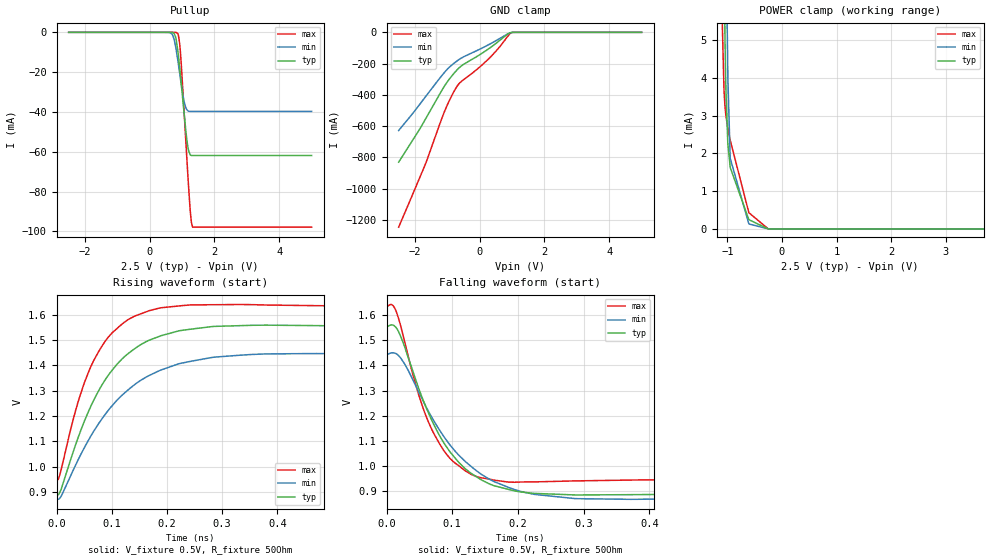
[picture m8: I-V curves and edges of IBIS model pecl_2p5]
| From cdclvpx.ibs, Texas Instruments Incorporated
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|   Pecl_2p5 Model   |
[Model]   pecl_2p5
Model_type   Open_source
Polarity   Non-Inverting
Vmeas = 1.22
Vref = 0.5
Cref = 1pF
Rref = 50
|   typ   min   max
|   (nom PVT)   (fast PVT)   (slow PVT)
C_comp   1.172e-13   1.121e-13   1.238e-13
[Model Spec]
|Subparameter
Vmeas   1.22V   1.16V   1.3V
| Vmeas is the expected cross point for each differential signal pair.
| Where nom  PVT is Nominal Process, 2.5V, 40C
|   Fast PVT is Strong Process,  2.625V, -40C
|   Slow PVT is Weak Process,   2.375V,100C
[Voltage Range]   2.5   2.375   2.625
|Junction Temperature
[Temperature range]   40   100   -40
[Pullup Reference]   2.5   2.375   2.625
[Pulldown Reference]   0   0   0
[Power Clamp Reference]   2.5   2.375   2.625
[GND Clamp Reference]   0   0   0
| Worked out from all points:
|   falling waveform, V_fixture 0.5V, R_fixture 50Ohm: 20-80 % time 72.8ps typ, 91.4ps min, 54.2ps max; typ from 1.55 V to 0.89 V
|   rising waveform, V_fixture 0.5V, R_fixture 50Ohm: 20-80 % time 91.7ps typ, 114ps min, 69.7ps max; typ from 0.89 V to 1.55 V
[GND Clamp]
|   Voltage   I(typ)   I(min)   I(max)
-2.5V     -829.8mA   -627.6mA   -1.246A
-1.827V   -610.9mA   -454.4mA   -917.9mA
-1.655V   -548.5mA   -407.4mA   -833.1mA
-1.09V    -345.1mA   -257.2mA   -508.6mA
-932.9mV  -298.3mA   -222.7mA   -434.9mA
-770mV    -256.8mA   -194.2mA   -369.5mA
-621.4mV  -224.8mA   -171.9mA   -324.6mA
-79.75mV  -153.8mA   -116.3mA   -236.2mA
352.4mV   -94.38mA   -70.87mA   -154mA
950mV     -2.212mA   -3.472mA   -5.936mA
1.078V    -34.58uA   -148.2uA   -28.47uA
5V        0A         0A         0A
[Pullup]
|   Voltage   I(typ)   I(min)   I(max)
-2.5V     0A         0A         0A
650mV     -16.5uA    -287.6uA   -23.75nA
799.6mV   -2.244mA   -6.925mA   -26.92uA
870mV     -9.197mA   -14.07mA   -689.7uA
928.3mV   -17.88mA   -20.73mA   -5.854mA
950.9mV   -21.58mA   -23.37mA   -10.13mA
1.06V     -40mA      -34.6mA    -38.68mA
1.167V    -56.25mA   -39.23mA   -68.43mA
1.251V    -61.52mA   -39.72mA   -89.32mA
1.288V    -61.88mA   -39.72mA   -95.39mA
1.33V     -61.88mA   -39.72mA   -97.87mA
5V        -61.88mA   -39.72mA   -97.87mA
[POWER Clamp]
|   Voltage   I(typ)   I(min)   I(max)
-2.5V     661mA      670.7mA    652.1mA
-1.093V   12.53mA    22.3mA     5.341mA
-1.063V   7.208mA    14.74mA    3.688mA
-1.046V   5.126mA    11.09mA    3.26mA
-1.032V   4.003mA    8.755mA    3.053mA
-1.027V   3.66mA     7.959mA    2.989mA
-992.5mV  2.258mA    4.039mA    2.663mA
-991.9mV  2.243mA    3.989mA    2.658mA
-949.1mV  1.628mA    1.87mA     2.348mA
-607.4mV  245.3uA    132.7uA    430.7uA
-250mV    157.5nA    146.5nA    75.55nA
5V        0A         0A         0A
[Ramp]
R_load = 50
|   typ   min   max
dV/dt_r   0.3974/9.16262e-11   0.341435/1.13903e-10   0.411413/6.97887e-11
dV/dt_f   0.397382/7.28052e-11   0.341442/9.13749e-11   0.411378/5.41457e-11
[Falling Waveform]
V_fixture = 0.5V
V_fixture_min = 0.375V
V_fixture_max = 0.625V
R_fixture = 50Ohm
|   Time   V(typ)   V(min)   V(max)
0s        1.552V     1.442V     1.633V
7.8ps     1.561V     1.45V      1.642V
14.6ps    1.55V      1.446V     1.616V
49ps      1.308V     1.295V     1.283V
72.2ps    1.163V     1.179V     1.128V
97.2ps    1.054V     1.082V     1.029V
137.4ps   956.2mV    980mV      957.6mV
203.4ps   896.9mV    899.4mV    936.2mV
287ps     884.9mV    870.4mV    940.7mV
843.8ps   890.1mV    873mV      947.1mV
[Rising Waveform]
V_fixture = 0.5V
V_fixture_min = 0.375V
V_fixture_max = 0.625V
R_fixture = 50Ohm
|   Time   V(typ)   V(min)   V(max)
0s        890mV      873mV      947mV
8.4ps     910.9mV    883.1mV    987.9mV
40ps      1.12V      1.031V     1.262V
68ps      1.265V     1.142V     1.421V
102ps     1.384V     1.244V     1.53V
131.6ps   1.449V     1.306V     1.583V
166.8ps   1.498V     1.358V     1.614V
222.6ps   1.536V     1.406V     1.634V
354.2ps   1.558V     1.442V     1.639V
893.4ps   1.552V     1.442V     1.633V
